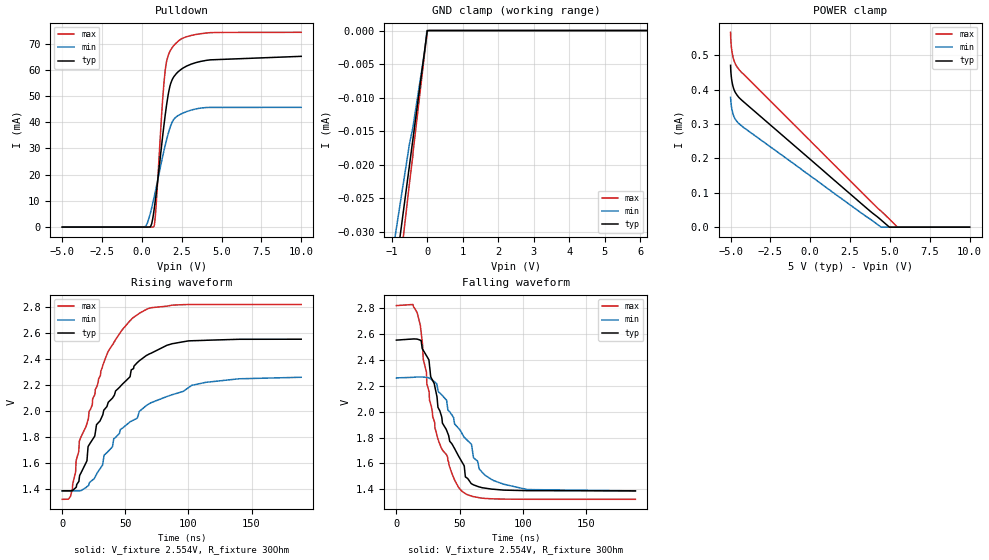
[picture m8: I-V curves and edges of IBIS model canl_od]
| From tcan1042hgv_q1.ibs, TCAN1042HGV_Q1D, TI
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|   canl_od Model
[Model]   canl_od
Model_type   I/O_open_drain
Polarity   Non-Inverting
Enable   Active-Low
Vinl = 0.5
Vinh = 0.9
Vmeas = 2
Vref = 2.554
Cref = 2pF
Rref = 30
|   typ   min   max
|   (nom PVT)   (fast PVT)   (slow PVT)
C_comp   9.866e-12   9.101e-12   1.128e-11
| Where nom  PVT is Nominal Process, 5V, 27C
|   Fast PVT is Strong Process,  5.5V, -55C
|   Slow PVT is Weak Process,   4.5V, 150C
[Voltage Range]   5   4.5   5.5
|Junction Temperature
[Temperature Range]   27   150   -55
[Pullup Reference]   5   4.5   5.5
[Pulldown Reference]   0   0   0
[Power Clamp Reference]   5   4.5   5.5
[GND Clamp Reference]   0   0   0
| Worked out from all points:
|   slope of the pulldown table from 0 to 0.75 V, typ, clamps not added: 126 ohm
|   falling waveform, V_fixture 2.554V, R_fixture 30Ohm: 20-80 % time 24.7ns typ, 25.7ns min, 20.1ns max; typ from 2.55 V to 1.39 V
|   rising waveform, V_fixture 2.554V, R_fixture 30Ohm: 20-80 % time 35.5ns typ, 45.6ns min, 29.5ns max; typ from 1.39 V to 2.55 V
[Pulldown]
|   Voltage   I(typ)   I(min)   I(max)
-5V       -98.49uA   -74.66uA   -125.6uA
175mV     -96.5uA    1.755uA    -123.6uA
545mV     109.6uA    5.535mA    -119.8uA
747.5mV   5.728mA    10.77mA    70.23uA
854.5mV   10.59mA    13.79mA    4.945mA
1.286V    33.79mA    26.45mA    47.23mA
1.485V    43.73mA    31.74mA    60.85mA
1.633V    49.9mA     35.24mA    65.2mA
1.809V    54.86mA    38.69mA    67.69mA
2.295V    59.42mA    42.64mA    71.12mA
4.091V    63.71mA    45.65mA    74.16mA
10V       65.21mA    45.69mA    74.39mA
[GND Clamp]
|   Voltage   I(typ)   I(min)   I(max)
-5V       -201.8uA   -172.1uA   -233.7uA
-3.794V   -152.1uA   -129.3uA   -175.4uA
-495.5mV  -20.08uA   -16.88uA   -22.74uA
-405mV    -16.46uA   -14.59uA   -18.83uA
-401mV    -16.3uA    -14.49uA   -18.83uA
-396.5mV  -16.12uA   -14.32uA   -18.22uA
-59mV     -2.587uA   -2.802uA   -2.961uA
-5mV      -422.6nA   0A         -608.7nA
5mV       -21.85nA   0A         0A
10V       0A         0A         0A
[POWER Clamp]
|   Voltage   I(typ)   I(min)   I(max)
-5V       471uA      378.2uA    567.2uA
-4.995V   464.8uA    373.9uA    556.9uA
-4.984V   454.6uA    368.2uA    544.7uA
-4.95V    436.8uA    353.6uA    524.9uA
-4.895V   419.6uA    338.2uA    506.3uA
-4.84V    408.8uA    328.7uA    493.8uA
-4.697V   391.7uA    313.7uA    474.6uA
-4.466V   377uA      301.2uA    458.2uA
4.45V     20.82uA    56.11nA    46.65uA
4.97V     32.32nA    0A         23.29uA
5.472V    0A         0A         87.45nA
10V       0A         0A         0A
[Ramp]
R_load = 30
|   typ   min   max
dV/dt_r   0.699535/3.55292e-08   0.524436/4.53315e-08   0.898885/2.95412e-08
dV/dt_f   0.699494/2.47352e-08   0.524499/2.56416e-08   0.89889/2.01117e-08
[Falling Waveform]
V_fixture = 2.554V
V_fixture_min = 2.262V
V_fixture_max = 2.821V
R_fixture = 30Ohm
|   Time   V(typ)   V(min)   V(max)
0s        2.554V     2.262V     2.821V
16.46ns   2.562V     2.268V     2.766V
25.79ns   2.4V       2.261V     2.158V
31.98ns   2.124V     2.215V     1.818V
36.49ns   1.911V     2.124V     1.704V
52.33ns   1.605V     1.825V     1.382V
59.3ns    1.444V     1.75V      1.349V
65.65ns   1.418V     1.557V     1.335V
85.02ns   1.394V     1.44V      1.324V
189.3ns   1.388V     1.388V     1.323V
[Rising Waveform]
V_fixture = 2.554V
V_fixture_min = 2.262V
V_fixture_max = 2.821V
R_fixture = 30Ohm
|   Time   V(typ)   V(min)   V(max)
0s        1.388V     1.388V     1.323V
6.618ns   1.388V     1.388V     1.346V
10.62ns   1.412V     1.388V     1.534V
10.98ns   1.415V     1.388V     1.62V
13.57ns   1.491V     1.388V     1.772V
27.17ns   1.897V     1.515V     2.185V
35.36ns   2.036V     1.681V     2.437V
56.33ns   2.327V     1.932V     2.721V
102.4ns   2.542V     2.198V     2.82V
189.3ns   2.554V     2.261V     2.821V
